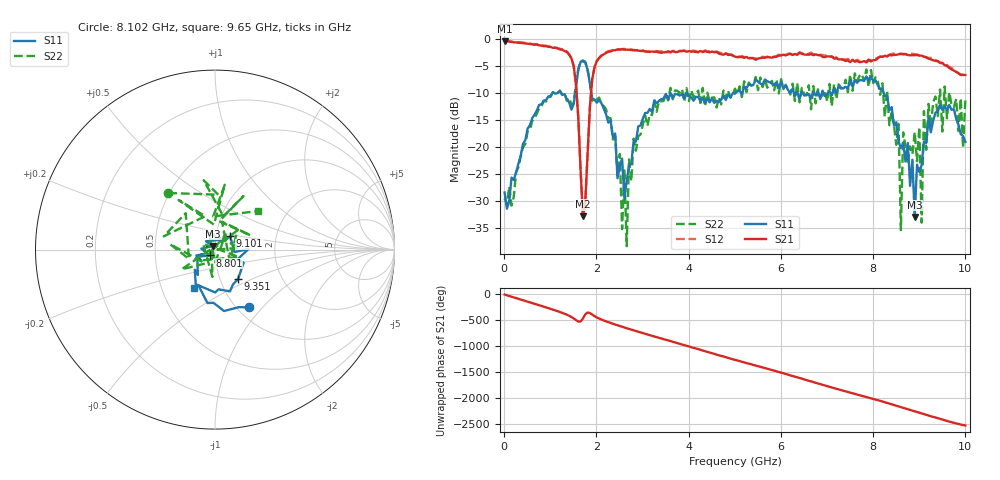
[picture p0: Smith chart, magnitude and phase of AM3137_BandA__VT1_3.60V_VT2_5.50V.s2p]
! Date/Time: Tue, Nov 13, 2018 4:48 PM
! Network Analyzer: Agilent Technologies E8364B Rev: A.07.50.67
! Sweep from 0.010 to 10.000 GHz, 201 Points, Sweep Type: LIN
! Power Supply: 3.601 V, -0.004 A
# Hz S DB R 50
!freq MagS11 AngS11 MagS21 AngS21 MagS12 AngS12 MagS22 AngS22
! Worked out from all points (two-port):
!   201 points, 10 MHz to 10 GHz, reference 50 ohm
!   highest |S21| = -0.34 dB at 10 MHz (marker M1); lowest = -32.8 dB at 1.708 GHz (marker M2)
!   |S21| within 3 dB of the highest: start of sweep to 1.445 GHz; 2.076 GHz to 5.178 GHz (3.101 GHz wide, 85.5 % of centre)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
!   lowest |S11| = -32.9 dB at 8.901 GHz (marker M3), VSWR 1.05, Z = 48.9 + j1.95 ohm
!   |S11| at or under -10 dB: start of sweep to 1.044 GHz; 1.891 GHz to 3.604 GHz (1.713 GHz wide, 62.3 % of centre); 8.231 GHz to end of sweep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
!   |S22| runs from -38.4 to -4.0 dB; largest |S21 - S12| = 0.032
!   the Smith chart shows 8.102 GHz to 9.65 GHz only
!   S11 on the Smith chart (normalised r, x): 8.102 GHz: 1.13, -0.85; 8.801 GHz: 0.94, -0.06; 9.101 GHz: 1.17, +0.18; 9.351 GHz: 1.22, -0.42; 9.65 GHz: 0.72, -0.33
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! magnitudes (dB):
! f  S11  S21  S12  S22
! 10 MHz  -28.4  -0.3  -0.2  -29.5
! 1.459 GHz  -13.0  -3.5  -3.5  -12.1
! 1.708 GHz  -3.9  -32.8  -33.0  -4.1
! 1.958 GHz  -11.2  -5.2  -5.2  -10.9
! 2.657 GHz  -26.3  -1.9  -1.8  -38.4
! 2.807 GHz  -19.0  -2.0  -2.0  -18.4
! 3.357 GHz  -11.4  -2.4  -2.2  -11.4
! 5.005 GHz  -10.1  -3.2  -3.0  -9.1
! 6.703 GHz  -9.9  -2.9  -2.8  -8.7
! 8.102 GHz  -8.5  -3.5  -3.4  -7.8
! 8.352 GHz  -13.1  -2.9  -2.8  -15.9
! 8.551 GHz  -19.0  -2.8  -2.7  -15.7
! 8.601 GHz  -20.1  -2.7  -2.7  -35.4
! 8.651 GHz  -19.3  -2.7  -2.8  -17.3
! 8.801 GHz  -27.2  -3.0  -2.7  -19.9
! 8.901 GHz  -32.9  -2.9  -2.8  -17.2
! 9.001 GHz  -24.6  -3.0  -3.0  -16.3
! 9.051 GHz  -23.4  -3.0  -3.0  -34.0
! 9.101 GHz  -19.0  -3.2  -3.2  -13.3
! 9.351 GHz  -13.6  -4.0  -3.9  -10.6
! 9.65 GHz  -12.2  -5.3  -5.1  -9.8
! 10 GHz  -19.0  -6.6  -6.5  -11.0
